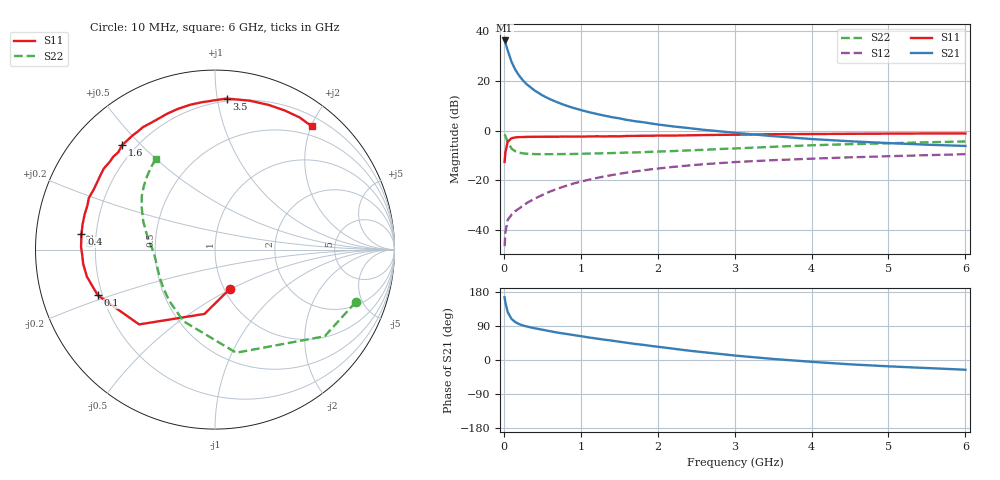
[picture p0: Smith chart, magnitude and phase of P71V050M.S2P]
! SIEMENS Small Signal Semiconductors
! BFP196
! Si NPN RF Bipolar Junction Transistor in SOT143
! VCE = 1 V  IC = 50 mA
! Common Emitter S-Parameters:  May  1996
# GHz  S  MA  R  50
!  f  S11  S21  S12  S22
! GHz  MAG  ANG  MAG  ANG  MAG  ANG  MAG  ANG
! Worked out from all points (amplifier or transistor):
!   36 points, 10 MHz to 6 GHz, reference 50 ohm
!   highest |S21| = 36.1 dB at 10 MHz (marker M1)
!   |S21| within 3 dB of that: start of sweep to 40.61 MHz
!   unconditionally stable (mu >= 1): 379.3 MHz to end of sweep
!   at 250 MHz: K = 0.89, MSG = 25.1 dB, |S12| = -30.1 dB
!   at 1.4 GHz: K = 1.11, MAG = 9.6 dB, |S12| = -17.9 dB
!   at 6 GHz: K = 1.02, MAG = 0.9 dB, |S12| = -9.5 dB
!   S11 on the Smith chart (normalised r, x): 10 MHz: 1.06, -0.49; 100 MHz: 0.18, -0.18; 400 MHz: 0.14, +0.06; 1.6 GHz: 0.15, +0.44; 3.5 GHz: 0.18, +1.06; 6 GHz: 0.35, +2.00
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0.01  0.2351 -69.7  64.07 165.5  0.0048 75.2  0.8369 -20.4
0.02  0.3632 -99.3  58.09 151.9  0.009 65.6  0.779 -38.3
0.05  0.5937 -135.4  40.52 126.5  0.0162 49.6  0.5866 -78.4
0.1  0.7008 -158.7  23.84 108.3  0.0205 45.2  0.4359 -113.8
0.15  0.7293 -168.0  16.48 99.9  0.0243 47.1  0.3827 -131.8
0.2  0.7387 -173.8  12.56 94.6  0.0275 50.8  0.3597 -142.6
0.25  0.7408 -177.9  10.05 91.0  0.0311 52.9  0.3485 -150.1
0.3  0.7464 178.8  8.419 88.3  0.0354 56.4  0.3429 -154.8
0.4  0.7491 173.3  6.361 83.8  0.043 59.3  0.3368 -161.7
0.5  0.7511 169.2  5.089 80.0  0.051 61.0  0.3357 -166.2
0.6  0.7524 165.0  4.252 76.0  0.0598 61.7  0.3356 -169.3
0.7  0.7522 160.8  3.664 72.2  0.0682 61.8  0.3366 -171.6
0.9  0.7545 154.0  2.856 66.0  0.0861 60.8  0.339 -175.6
1.1  0.7609 147.1  2.35 59.7  0.1028 59.2  0.345 -178.4
1.3  0.7634 140.5  2.002 53.8  0.1196 56.6  0.3501 178.9
1.6  0.7788 131.7  1.634 45.5  0.1436 52.3  0.3612 175.4
2.2  0.7924 115.0  1.21 29.9  0.1865 43.3  0.3876 167.8
2.8  0.8187 99.7  0.968 16.2  0.2222 34.1  0.4258 159.3
3.5  0.8443 85.6  0.772 2.8  0.2545 24.0  0.4721 149.9
4.5  0.8598 69.6  0.609 -11.4  0.2901 11.8  0.5328 138.0
5.5  0.8742 57.4  0.52 -21.2  0.3208 1.0  0.5809 127.9
6  0.8733 52.0  0.491 -25.7  0.3353 -4.7  0.6039 123.0
